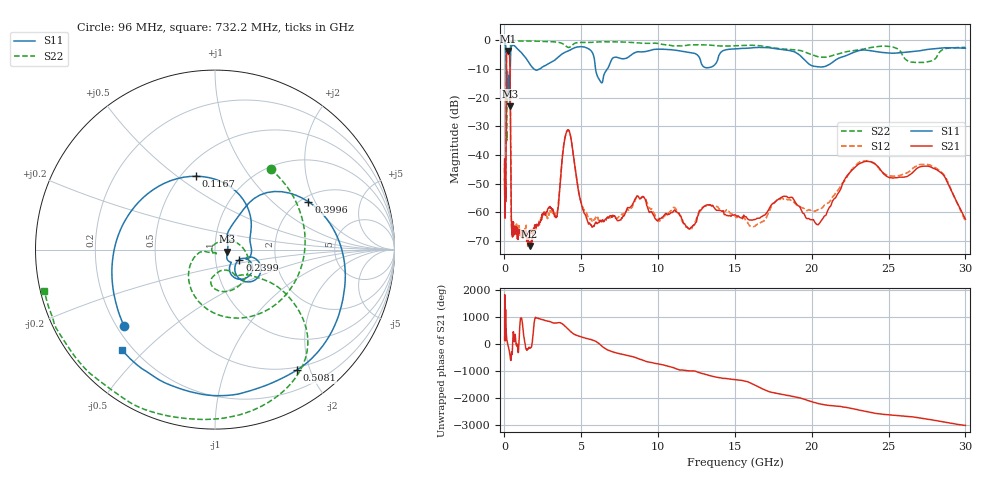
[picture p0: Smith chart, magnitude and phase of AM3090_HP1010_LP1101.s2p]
! Date/Time: Thu, Feb 28, 2019 2:04 PM
! Network Analyzer: Agilent Technologies E8364B Rev: A.07.50.67
! Sweep from 0.010 to 30.000 GHz, 1601 Points, Sweep Type: LOG
! Power Supply: 5.023 V, 0.002 A
# Hz S DB R 50
!freq MagS11 AngS11 MagS21 AngS21 MagS12 AngS12 MagS22 AngS22
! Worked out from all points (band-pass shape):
!   1601 points, 10 MHz to 30 GHz, reference 50 ohm
!   highest |S21| = -3.73 dB at 237.5 MHz (marker M1); lowest = -71.7 dB at 1.63 GHz (marker M2)
!   |S21| within 3 dB of the highest: 129.3 MHz to 347.7 MHz (218.4 MHz wide, 91.6 % of centre)
!   lowest |S11| = -23.1 dB at 340.5 MHz (marker M3), VSWR 1.15, Z = 57.4 - j1.34 ohm
!   |S11| at or under -10 dB: 122.2 MHz to 381.4 MHz (259.2 MHz wide, 103 % of centre); 1.9 GHz to 2.287 GHz (387.4 MHz wide, 18.5 % of centre); 5.927 GHz to 6.708 GHz (781.2 MHz wide, 12.4 % of centre)
!   |S22| runs from -35.2 to -0.1 dB; largest |S21 - S12| = 0.011
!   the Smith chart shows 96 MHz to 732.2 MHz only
!   S11 on the Smith chart (normalised r, x): 96 MHz: 0.23, -0.35; 116.7 MHz: 0.59, +0.59; 239.9 MHz: 1.30, -0.15; 399.6 MHz: 2.19, +1.77; 508.1 MHz: 0.46, -1.79; 732.2 MHz: 0.16, -0.43
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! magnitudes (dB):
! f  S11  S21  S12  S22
! 10 MHz  -0.2  -41.4  -44.6  -0.7
! 38.04 MHz  -0.5  -61.6  -57.6  -1.6
! 96 MHz  -3.6  -49.4  -47.1  -5.3
! 116.7 MHz  -7.5  -16.0  -16.0  -8.4
! 144.7 MHz  -14.0  -4.7  -4.7  -34.5
! 237.5 MHz  -16.9  -3.7  -3.7  -15.6
! 239.9 MHz  -16.7  -3.7  -3.7  -15.8
! 340.5 MHz  -23.1  -6.0  -6.0  -12.6
! 399.6 MHz  -4.7  -34.6  -34.7  -1.2
! 446.1 MHz  -2.3  -62.2  -62.4  -0.4
! 508.1 MHz  -1.8  -67.3  -63.8  -0.2
! 550.5 MHz  -1.8  -65.8  -67.6  -0.2
! 732.2 MHz  -2.4  -65.4  -67.8  -0.2
! 1.63 GHz  -8.2  -71.7  -67.4  -0.3
! 2.084 GHz  -10.5  -64.6  -64.7  -0.4
! 3.385 GHz  -6.4  -61.4  -60.7  -0.7
! 4.115 GHz  -3.8  -31.3  -31.3  -2.5
! 5.528 GHz  -3.2  -63.7  -61.9  -0.8
! 7.926 GHz  -6.3  -59.6  -59.7  -0.7
! 20.2 GHz  -9.1  -63.5  -59.7  -5.4
! 23.48 GHz  -3.5  -42.3  -42.1  -3.0
! 30 GHz  -2.8  -62.4  -63.1  -2.5
